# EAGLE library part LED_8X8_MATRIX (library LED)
CPD-15088A YGD2/A Green 8x8 LED matrix
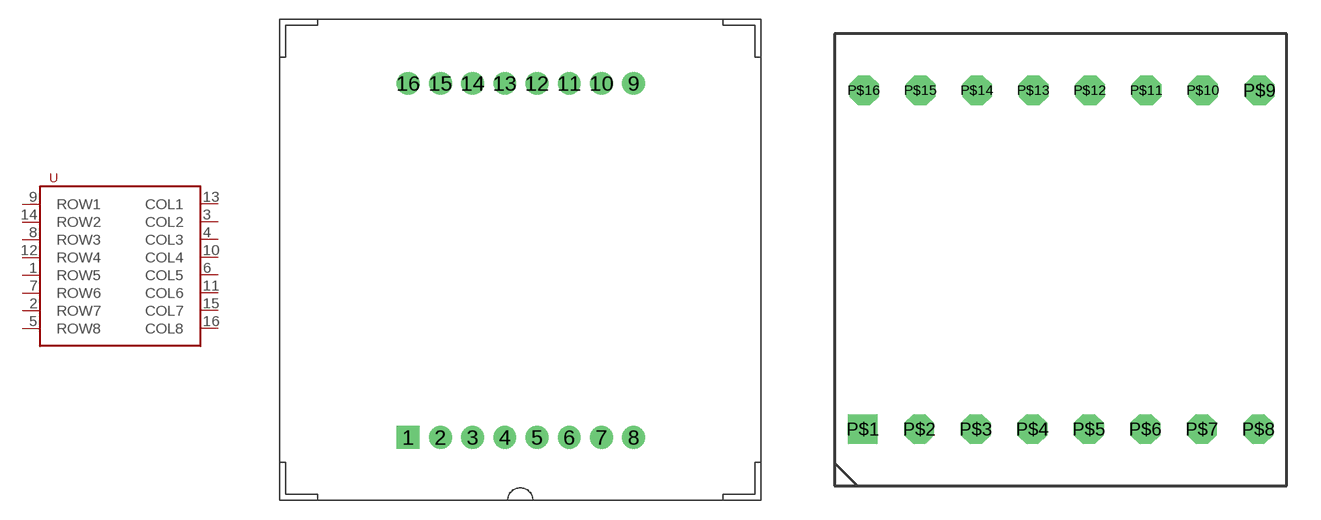
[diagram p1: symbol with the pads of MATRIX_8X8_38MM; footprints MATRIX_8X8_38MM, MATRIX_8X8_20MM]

Designator prefix -

## LED_8X8_MATRIXYGD2/A  [MATRIX_8X8_38MM]
1  ROW5
2  ROW7
3  COL2
4  COL3
5  ROW8
6  COL5
7  ROW6
8  ROW3
9  ROW1
10  COL4
11  COL6
12  ROW4
13  COL1
14  ROW2
15  COL7
16  COL8

## LED_8X8_MATRIX07088BH  [MATRIX_8X8_20MM]
P$1  ROW4
P$2  ROW2
P$3  COL2
P$4  COL3
P$5  ROW1
P$6  COL5
P$7  ROW3
P$8  ROW6
P$9  ROW8
P$10  COL4
P$11  COL6
P$12  ROW5
P$13  COL1
P$14  ROW7
P$15  COL7
P$16  COL8

## Footprint MATRIX_8X8_38MM (pad centres in mm)
CPD-15088 LED Matrix 8x8 38mm Green
drill 0.5 pad 1.8 square: 1 10.16,-33.02
drill 0.5 pad 1.8: 2 12.7,-33.02; 3 15.24,-33.02; 4 17.78,-33.02; 5 20.32,-33.02; 6 22.86,-33.02; 7 25.4,-33.02; 8 27.94,-33.02; 9 27.94,-5.08; 10 25.4,-5.08; 11 22.86,-5.08; 12 20.32,-5.08; 13 17.78,-5.08; 14 15.24,-5.08; 15 12.7,-5.08; 16 10.16,-5.08

## Footprint MATRIX_8X8_20MM (pad centres in mm)
LED Matrix 8x8 20mm RED 07088BH Rows - anodes
drill 0.8 square: P$1 1.25,2.5
drill 0.8 octagon: P$2 3.75,2.5; P$3 6.25,2.5; P$4 8.75,2.5; P$5 11.25,2.5; P$6 13.75,2.5; P$7 16.25,2.5; P$8 18.75,2.5; P$9 18.8,17.5; P$10 16.3,17.5; P$11 13.8,17.5; P$12 11.3,17.5; P$13 8.8,17.5; P$14 6.3,17.5; P$15 3.8,17.5; P$16 1.3,17.5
